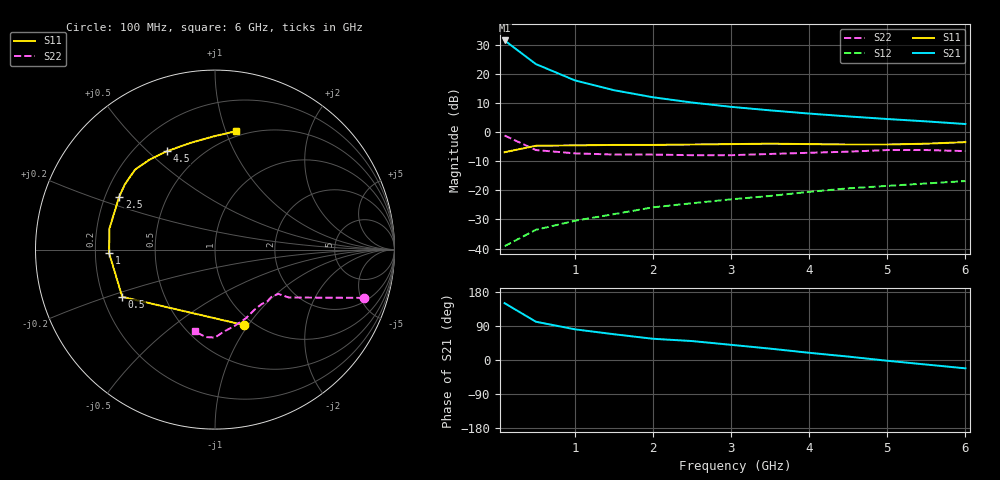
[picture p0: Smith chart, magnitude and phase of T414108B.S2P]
!AT-41410
!S-PARAMETERS at Vce=8V  Ic=25mA.  LAST UPDATED 07-21-92
# ghz s ma r 50
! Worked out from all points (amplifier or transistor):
!   13 points, 100 MHz to 6 GHz, reference 50 ohm
!   highest |S21| = 31.4 dB at 100 MHz (marker M1)
!   |S21| within 3 dB of that: start of sweep to 248.2 MHz
!   unconditionally stable (mu >= 1): 966.7 MHz to 5.277 GHz
!   at 1 GHz: K = 1.02, MAG = 23.2 dB, |S12| = -30.5 dB
!   at 3 GHz: K = 1.22, MAG = 13.0 dB, |S12| = -23.1 dB
!   at 6 GHz: K = 0.92, MSG = 9.8 dB, |S12| = -16.8 dB
!   S11 on the Smith chart (normalised r, x): 100 MHz: 0.91, -0.95; 500 MHz: 0.28, -0.22; 1 GHz: 0.26, -0.02; 2.5 GHz: 0.26, +0.24; 4.5 GHz: 0.33, +0.58; 6 GHz: 0.45, +1.09
0.1  0.45 -69.0  37.17 150.0  0.011 64.0  0.87 -18.0
0.5  0.58 -153.0  14.63 101.0  0.021 43.0  0.49 -33.0
1  0.59 -178.0  7.68 81.0  0.03 53.0  0.43 -35.0
1.5  0.6 169.0  5.21 68.0  0.039 58.0  0.41 -40.0
2  0.6 157.0  3.94 56.0  0.051 55.0  0.41 -45.0
2.5  0.61 151.0  3.2 50.0  0.06 55.0  0.4 -49.0
3  0.62 144.0  2.7 40.0  0.07 58.0  0.4 -56.0
3.5  0.63 135.0  2.35 30.0  0.08 54.0  0.42 -66.0
4  0.62 126.0  2.07 19.0  0.094 53.0  0.44 -76.0
4.5  0.61 116.0  1.85 9.0  0.108 45.0  0.46 -84.0
5  0.61 103.0  1.67 -2.0  0.119 41.0  0.49 -90.0
5.5  0.63 91.0  1.52 -12.0  0.131 34.0  0.49 -96.0
6  0.67 80.0  1.37 -22.0  0.144 29.0  0.47 -104.0
